TYPE STR_SEC_N107 :
STRUCT
	Output0_Flow_SP_7003_01					:	REAL	;
	Output0_Actuator_Control_7009_01		:	USINT	;
	Output0_Actuator_Position_SP_7009_02	:	REAL	;
	Output0_Ramp_Time_7008_01				:	UDINT	;
	Input0_Active_Exception_Status_F380_00	:	USINT	;
	Input0_Flow_Reading_6000_01				:	REAL	;
	Input0_Position_Setpoint_6009_01		:	REAL	;
END_STRUCT
END_TYPE
